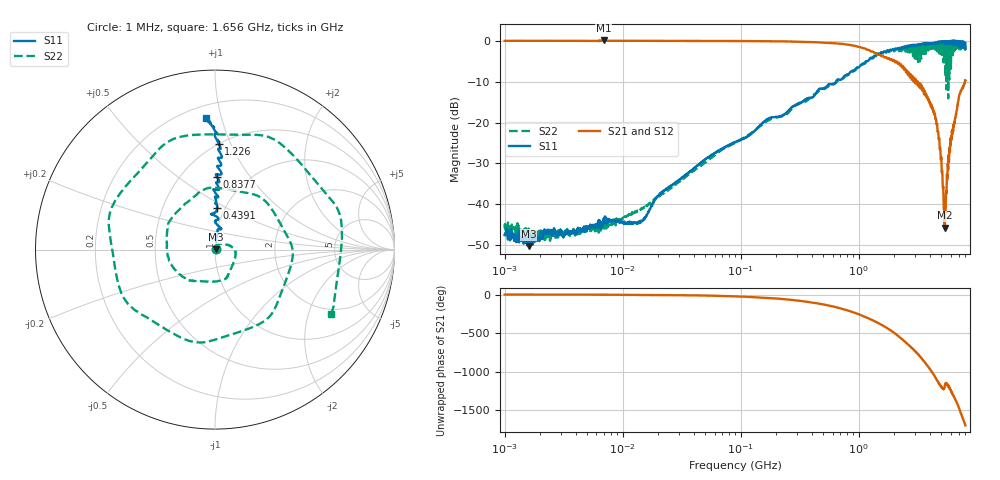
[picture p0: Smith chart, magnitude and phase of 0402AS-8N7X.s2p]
!s-Parameter Generated by FASTRON Sdn. Bhd.
!FASTRON P/N : 0402AS-8N7X
!Keysight Technologies: E5071C_MY46733604_B.14.02
!Date: Mon Dec 01 10:27:47 2025
!Version  :Rev00  Mon Dec 01 10:27:47 2025
!Data & Calibration Information:
!Freq  S11:SOLT2(ON)  S21:SOLT2(ON)  S12:SOLT2(ON)  S22:SOLT2(ON)
!PortZ  Port1:50+j0  Port2:50+j0
!When reading reference impedance value at option line is always used.
! Remarks : This data is being provided solely for informational purposes.
# Hz S dB R 50
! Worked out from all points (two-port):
!   1601 points, 1 MHz to 8 GHz, reference 50 ohm
!   highest |S21| = 0.04 dB at 6.912 MHz (marker M1); lowest = -45.7 dB at 5.332 GHz (marker M2)
!   |S21| within 3 dB of the highest: start of sweep to 1.353 GHz
!   lowest |S11| = -50.2 dB at 1.605 MHz (marker M3), VSWR 1.01, Z = 50.3 + j0.121 ohm
!   |S11| at or under -10 dB: start of sweep to 640.5 MHz
!   |S22| runs from -48.9 to -0.2 dB; largest |S21 - S12| = 0.021
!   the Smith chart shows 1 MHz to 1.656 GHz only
!   S11 on the Smith chart (normalised r, x): 1 MHz: 1.01, +0.00; 439.1 MHz: 0.92, +0.45; 837.7 MHz: 0.73, +0.71; 1.226 GHz: 0.50, +0.90; 1.656 GHz: 0.28, +0.89
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1000000  -47.50 13.0  -0.05 -0.3  -0.04 -0.3  -45.80 19.1
1604653  -50.20 22.9  -0.05 -0.4  -0.03 -0.5  -46.70 -4.1
4479405  -46.20 31.8  -0.05 -1.2  -0.04 -1.2  -46.60 39.8
6911657  -43.40 25.4  0.04 -2.2  -0.13 -1.9  -43.90 32.3
2.00676e7  -37.80 55.0  -0.05 -5.3  -0.05 -5.2  -38.10 66.6
8.994653e7  -24.80 87.3  -0.09 -23.5  -0.09 -23.4  -24.90 31.2
4.006501e8  -13.90 93.3  -0.34 -103.0  -0.34 -103.0  -13.60 -123.0
4.391133e8  -12.60 86.9  -0.41 -113.0  -0.40 -113.0  -12.80 -136.0
8.377436e8  -7.84 88.5  -1.05 145.0  -1.04 145.0  -8.14 21.6
1.225806e9  -4.59 88.0  -2.34 46.3  -2.34 46.2  -4.89 -178.0
1.434622e9  -3.29 91.0  -3.27 -4.7  -3.27 -4.8  -3.63 76.3
1.656419e9  -2.69 93.9  -4.13 -56.2  -4.13 -56.3  -2.60 -29.0
1.7949e9  -2.56 96.5  -4.26 -89.1  -4.26 -89.2  -2.73 -96.5
2.135779e9  -1.93 102.0  -5.62 -172.0  -5.62 -172.0  -1.90 92.1
2.486897e9  -1.57 108.0  -7.05 100.0  -7.03 100.0  -2.68 -89.0
2.853703e9  -1.40 114.0  -8.64 19.6  -8.60 19.4  -1.51 108.0
3.244011e9  -1.10 123.0  -10.40 -72.0  -10.30 -72.3  -1.46 -80.2
3.60885e9  -0.99 132.0  -12.30 -153.0  -12.30 -154.0  -1.06 92.6
3.973689e9  -0.64 137.0  -15.30 121.0  -15.30 120.0  -2.08 -84.7
4.324643e9  -0.77 142.0  -17.10 36.0  -17.10 35.4  -1.42 107.0
5.33235e9  -0.27 174.0  -45.70 -121.0  -45.70 -122.0  -5.71 -53.3
8e9  -0.56 -101.0  -9.70 102.0  -9.73 102.0  -2.28 141.0
